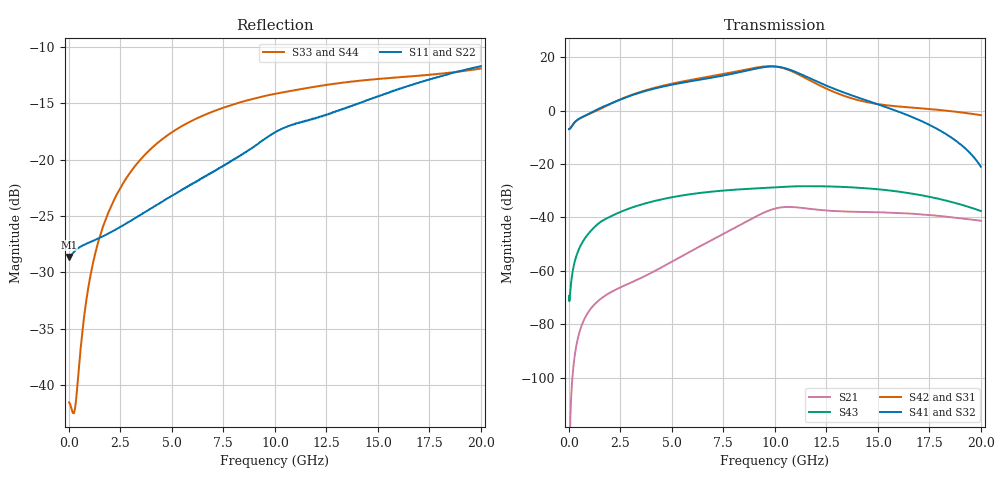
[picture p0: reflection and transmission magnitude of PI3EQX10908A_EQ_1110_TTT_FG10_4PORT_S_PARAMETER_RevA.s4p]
! NPort=4 DATA=2000 NOISE=0 GROUPDELAY=0 COMPLEX_DATAFORMAT=POLAR
! NumOfBlock=1 NumOfParam=0
! .MODEL Smodel S TSTONEFILE=PI3EQX10908A_EQ_1110_TTT_FG10_4PORT_S_PARAMETER_RevA.s4p TYPE=S
!  -- The above .MODEL line can be used for the S element in the netlist.
! The s parameter is extracted from the linear redriver, it is not bi-directional; only s(4,1)s(4,2) and s(3,1)s(3,2)
! should be the insertion loss
!Port definition:
!Port1 = input+
!Port2 = input-
!Port3 = output+
!Port4 = output-
# Hz S MA R  50
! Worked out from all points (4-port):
!   2000 points, 10 MHz to 20 GHz, reference 50 ohm
!   strongest paths, dB at 10 MHz, 5.01 GHz, 10.01 GHz, 15.01 GHz, 20 GHz:
!     S41: -6.9, 9.7, 16.5, 2.3, -21.0
!     S32: -6.9, 9.7, 16.5, 2.3, -21.0
!     S42: -6.9, 10.1, 16.5, 2.4, -1.7
!     S31: -6.9, 10.1, 16.5, 2.4, -1.7
!     S43: -69.4, -32.4, -28.7, -29.5, -37.6
!     S21: -127.2, -56.5, -36.7, -38.1, -41.2
!   lowest |S11| = -28.6 dB at 10 MHz (marker M1), VSWR 1.08, Z = 46.4 - j0.024 ohm
!   |S11| at or under -10 dB: start of sweep to end of sweep
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1e7  0.03701 -179.6  4.34e-07 14.6  0 0.0  0 0.0
     4.34e-07 14.6  0.03701 -179.6  0 0.0  0 0.0
     0.4506 1.2  0.4506 -178.8  0.008374 26.0  0.00034 -27.1
     0.4506 -178.8  0.4506 1.2  0.00034 -27.1  0.008374 26.0
6.37e9  0.0817 -121.3  0.002887 133.6  2.887e-07 68.8  1.617e-07 139.9
        0.002887 133.6  0.08173 -121.3  1.618e-07 139.9  2.887e-07 68.8
        4.033 -48.3  3.798 125.4  0.1549 15.2  0.02872 20.4
        3.798 125.5  4.033 -48.3  0.02872 20.4  0.1549 15.2
8.94e9  0.1137 -112.1  0.009737 108.9  2.146e-06 22.8  1.362e-06 113.9
        0.009739 108.9  0.1137 -112.1  1.362e-06 113.9  2.146e-06 22.8
        6.236 -111.4  5.961 62.8  0.1865 -5.4  0.03467 -6.4
        5.962 62.8  6.237 -111.4  0.03467 -6.4  0.1865 -5.4
1.026e10  0.1362 -112.3  0.01532 71.7  3.931e-06 -11.6  4.117e-06 80.4
          0.01532 71.7  0.1363 -112.3  4.117e-06 80.4  3.931e-06 -11.6
          6.468 -165.3  6.501 8.2  0.1981 -14.4  0.03715 -19.8
          6.502 8.2  6.468 -165.3  0.03715 -19.8  0.1981 -14.4
1.141e10  0.1478 -113.6  0.01491 40.6  4.98e-06 -22.6  7.371e-06 43.8
          0.01491 40.6  0.1479 -113.6  7.372e-06 43.8  4.98e-06 -22.6
          4.208 152.7  4.519 -37.0  0.2069 -21.0  0.0384 -33.4
          4.519 -37.0  4.208 152.7  0.0384 -33.4  0.2069 -21.0
1.36e10  0.1713 -112.0  0.01282 13.5  1.368e-05 -35.9  1.631e-05 -5.8
         0.01282 13.5  0.1714 -112.0  1.631e-05 -5.8  1.368e-05 -35.9
         1.758 122.1  2.01 -84.9  0.2216 -32.5  0.03678 -59.9
         2.01 -84.9  1.758 122.1  0.03678 -59.9  0.2216 -32.5
2e10  0.2602 -115.0  0.008669 -39.9  8.807e-05 -148.1  7.158e-05 -139.5
      0.008671 -39.9  0.2603 -115.0  7.158e-05 -139.5  8.806e-05 -148.1
      0.8211 52.6  0.08874 169.2  0.2539 -52.3  0.01318 -136.5
      0.0889 169.3  0.8213 52.6  0.01318 -136.5  0.2539 -52.3
